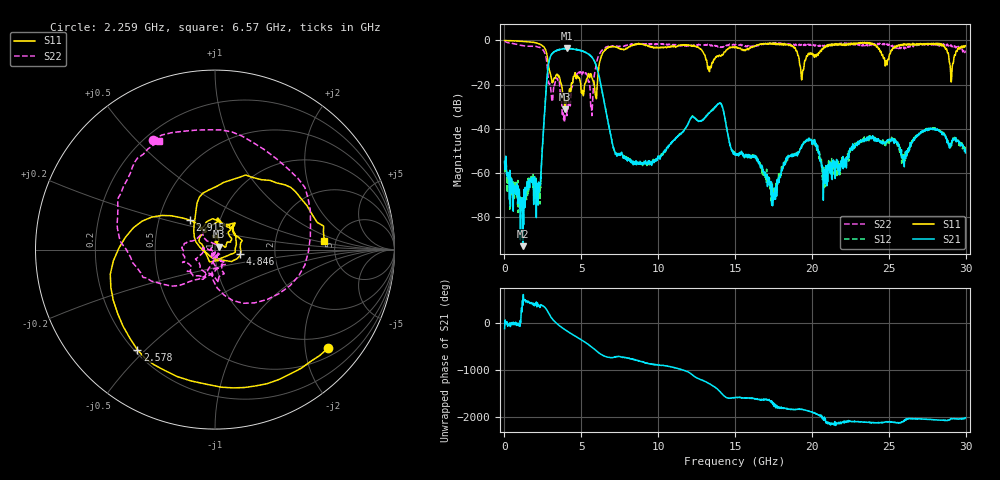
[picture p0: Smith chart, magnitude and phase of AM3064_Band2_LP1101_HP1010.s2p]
# Hz S DB R 50.0
!freq dBS11 angS11 dBS21 angS21 dBS12 angS12 dBS22 angS22
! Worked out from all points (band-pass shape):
!   1600 points, 10 MHz to 29.98 GHz, reference 50 ohm
!   highest |S21| = -3.61 dB at 4.059 GHz (marker M1); lowest = -93.3 dB at 1.191 GHz (marker M2)
!   |S21| within 3 dB of the highest: 3.038 GHz to 5.542 GHz (2.505 GHz wide, 58.4 % of centre)
!   lowest |S11| = -31.2 dB at 3.927 GHz (marker M3), VSWR 1.06, Z = 52.3 + j1.64 ohm
!   |S11| at or under -10 dB: 2.837 GHz to 6.189 GHz (3.352 GHz wide, 74.3 % of centre); 13.17 GHz to 13.5 GHz (331.5 MHz wide, 2.49 % of centre); 19.19 GHz to 19.51 GHz (325.5 MHz wide, 1.68 % of centre)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
!   |S22| runs from -37.0 to -0.2 dB; largest |S21 - S12| = 0.021
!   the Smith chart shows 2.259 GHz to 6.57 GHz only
!   S11 on the Smith chart (normalised r, x): 2.259 GHz: 0.69, -2.51; 2.578 GHz: 0.21, -0.47; 2.915 GHz: 0.72, +0.25; 4.846 GHz: 1.33, -0.07; 6.57 GHz: 4.05, +0.59
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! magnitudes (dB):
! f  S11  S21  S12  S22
! 10 MHz  0.0  -54.9  -54.7  -0.2
! 1.191 GHz  -0.5  -93.3  -85.1  -2.4
! 2.259 GHz  -1.6  -66.3  -64.0  -3.1
! 2.578 GHz  -3.0  -36.1  -36.1  -5.1
! 2.915 GHz  -13.4  -9.0  -8.9  -19.8
! 3.927 GHz  -31.2  -3.8  -3.6  -33.9
! 4.059 GHz  -27.6  -3.6  -3.7  -34.1
! 4.846 GHz  -16.9  -4.4  -4.4  -14.4
! 5.015 GHz  -23.8  -4.8  -4.6  -15.8
! 5.671 GHz  -16.8  -7.6  -7.4  -31.6
! 6.57 GHz  -4.3  -31.0  -30.9  -3.3
! 7.283 GHz  -3.1  -51.5  -50.7  -2.7
! 10 GHz  -3.4  -52.3  -53.2  -1.8
! 13.97 GHz  -6.7  -28.6  -28.5  -2.8
! 15 GHz  -3.0  -52.0  -51.9  -1.8
! 17.52 GHz  -1.5  -72.2  -70.2  -1.3
! 19.99 GHz  -5.8  -45.4  -45.3  -1.8
! 20.87 GHz  -2.6  -62.6  -58.4  -2.7
! 25 GHz  -8.4  -44.9  -45.1  -1.7
! 28.28 GHz  -1.4  -41.1  -41.1  -2.6
! 29.08 GHz  -17.5  -47.6  -46.2  -2.6
! 29.98 GHz  -2.4  -51.0  -50.0  -4.6
